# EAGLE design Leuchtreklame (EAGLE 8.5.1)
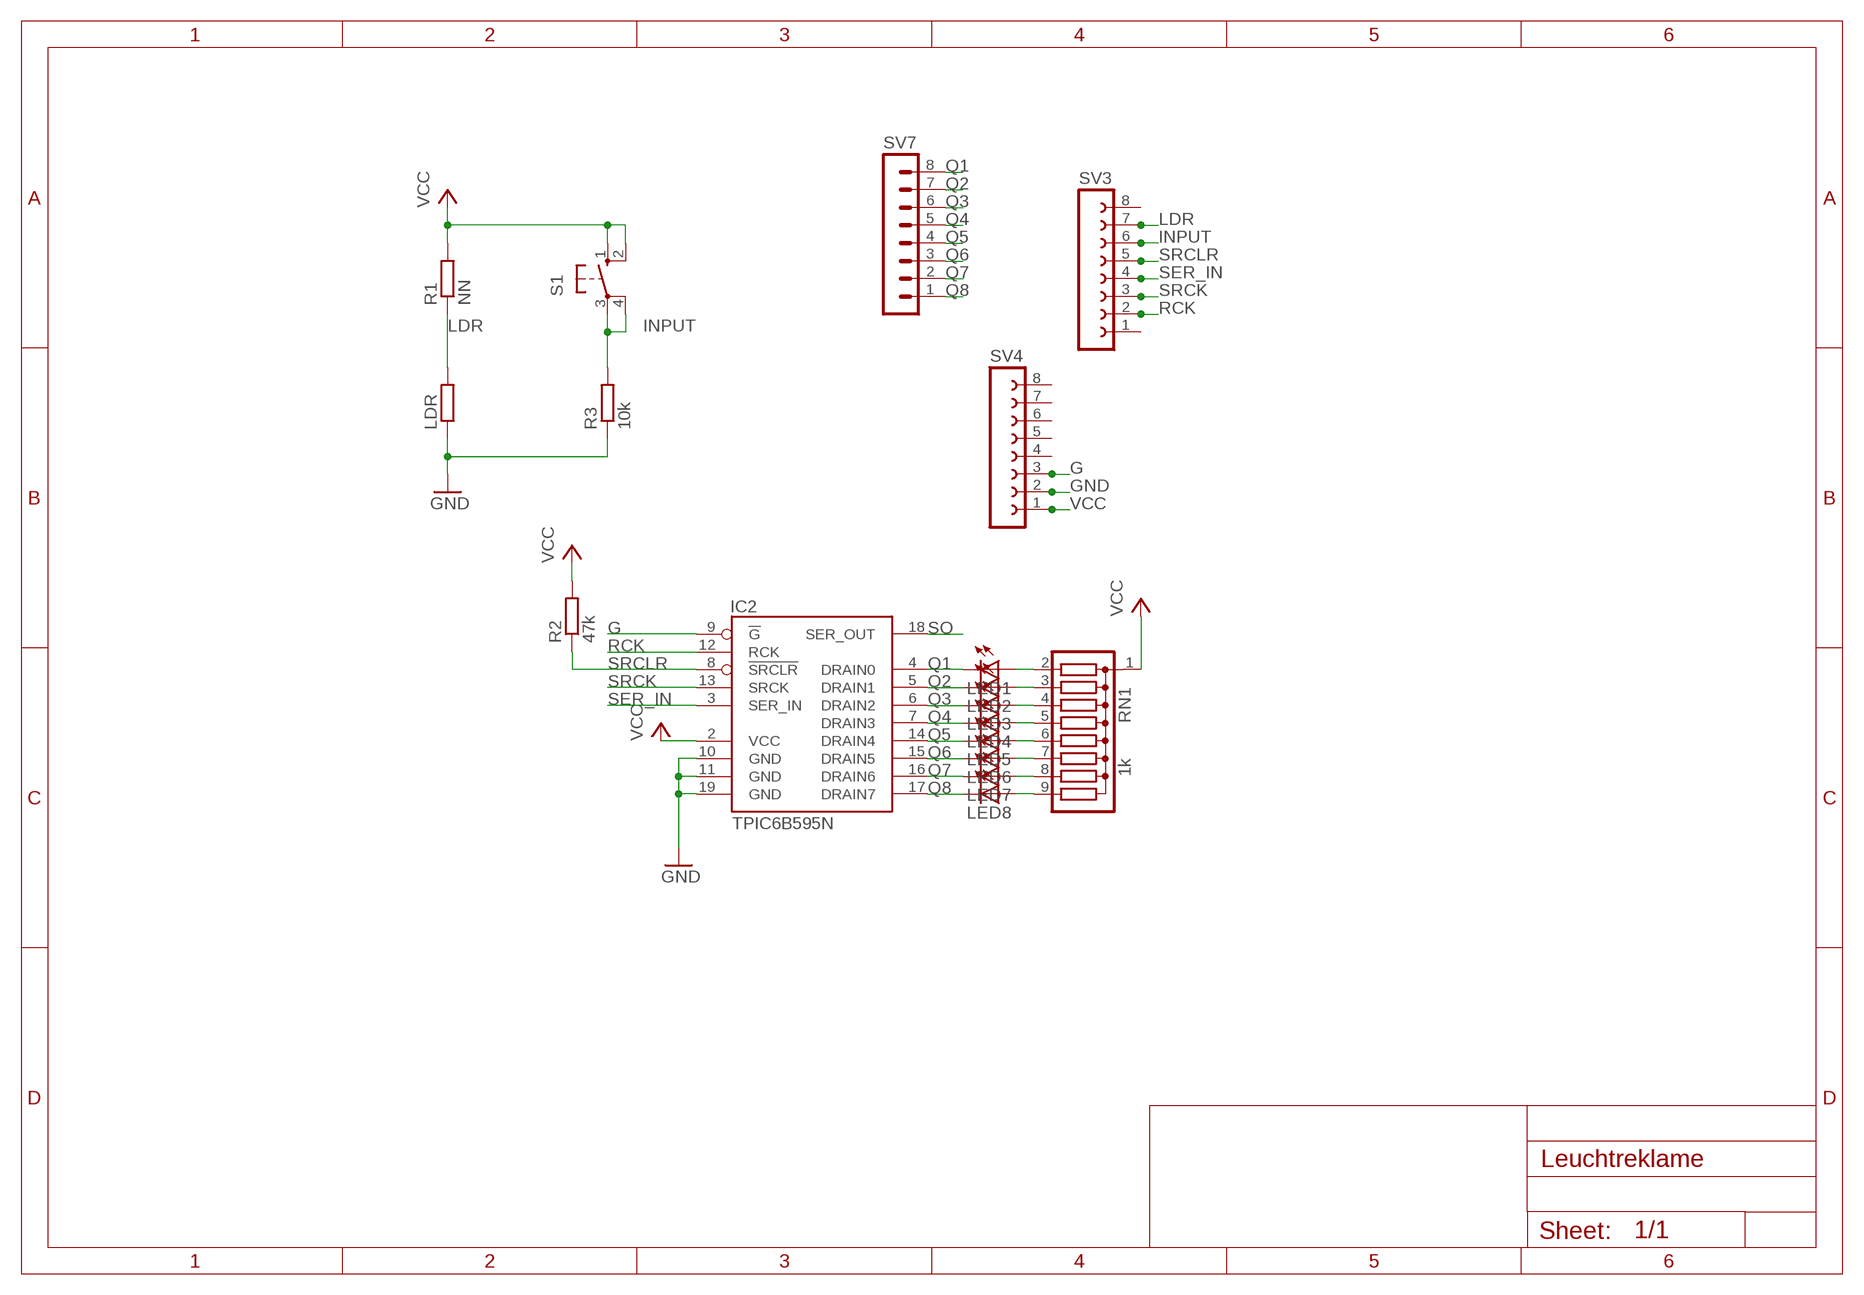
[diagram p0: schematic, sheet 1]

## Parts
IC2  TPIC6B595N  [DIL20]
LDR  R-EU_0204/5  [0204/5]
LED1  LEDSML0805  [SML0805]
LED2  LEDSML0805  [SML0805]
LED3  LEDSML0805  [SML0805]
LED4  LEDSML0805  [SML0805]
LED5  LEDSML0805  [SML0805]
LED6  LEDSML0805  [SML0805]
LED7  LEDSML0805  [SML0805]
LED8  LEDSML0805  [SML0805]
R1  NN  R-EU_0207/10  [0207/10]
R2  47k  R-EU_0207/10  [0207/10]
R3  10k  R-EU_0207/10  [0207/10]
RN1  1k  G08R  [SIL9]
S1  10-XX  [B3F-10XX]
SV3  FE08-1  [FE08]
SV4  FE08-1  [FE08]
SV7  MA08-1  [MA08-1]

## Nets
G: IC2.9(!G) SV4.3
GND: IC2.10(GND) IC2.11(GND) IC2.19(GND) LDR.1 R3.1 SV4.2
INPUT: R3.2 S1.3(P) S1.4(P1) SV3.6
LDR: LDR.2 R1.1 SV3.7
N$2: LED1.A RN1.2
N$3: LED2.A RN1.3
N$5: LED3.A RN1.4
N$6: LED4.A RN1.5
N$7: LED5.A RN1.6
N$8: LED6.A RN1.7
N$9: LED7.A RN1.8
N$10: LED8.A RN1.9
Q1: IC2.4(DRAIN0) LED1.C SV7.8
Q2: IC2.5(DRAIN1) LED2.C SV7.7
Q3: IC2.6(DRAIN2) LED3.C SV7.6
Q4: IC2.7(DRAIN3) LED4.C SV7.5
Q5: IC2.14(DRAIN4) LED5.C SV7.4
Q6: IC2.15(DRAIN5) LED6.C SV7.3
Q7: IC2.16(DRAIN6) LED7.C SV7.2
Q8: IC2.17(DRAIN7) LED8.C SV7.1
RCK: IC2.12(RCK) SV3.2
SER_IN: IC2.3(SER_IN) SV3.4
SO: IC2.18(SER_OUT)
SRCK: IC2.13(SRCK) SV3.3
SRCLR: IC2.8(!SRCLR) R2.1 SV3.5
VCC: IC2.2(VCC) R1.2 R2.2 RN1.1 S1.1(S) S1.2(S1) SV4.1
Unconnected: SV3.1 SV3.8 SV4.4 SV4.5 SV4.6 SV4.7 SV4.8

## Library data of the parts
IC2 = TPIC6B595:TPIC6B595
LDR R1-R3 = 1a BK_Hennef:R-EU_: RESISTOR, European symbol
LED1-LED8 = 1a BK_Hennef:LED: LED
RN1 = resistor-sil:G08R: SIL RESISTOR; OC_FARNELL: unknown; OC_NEWARK: unknown
S1 = switch-omron:10-XX: OMRON SWITCH; MPN: B3F-1000; OC_FARNELL: 176432; OC_NEWARK: 36M3542
SV3 SV4 = con-lsta:FE08-1: FEMALE HEADER; OC_FARNELL: unknown; OC_NEWARK: unknown
SV7 = con-lstb:MA08-1: PIN HEADER; OC_FARNELL: unknown; OC_NEWARK: unknown

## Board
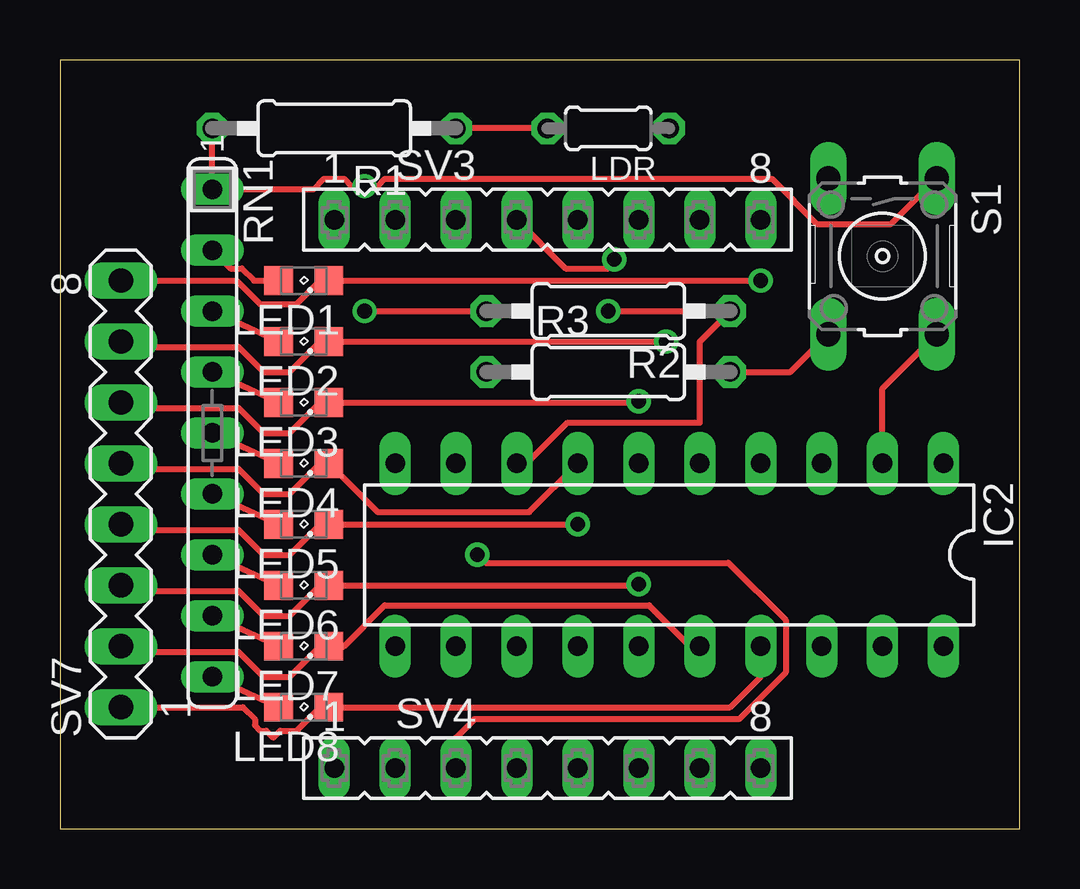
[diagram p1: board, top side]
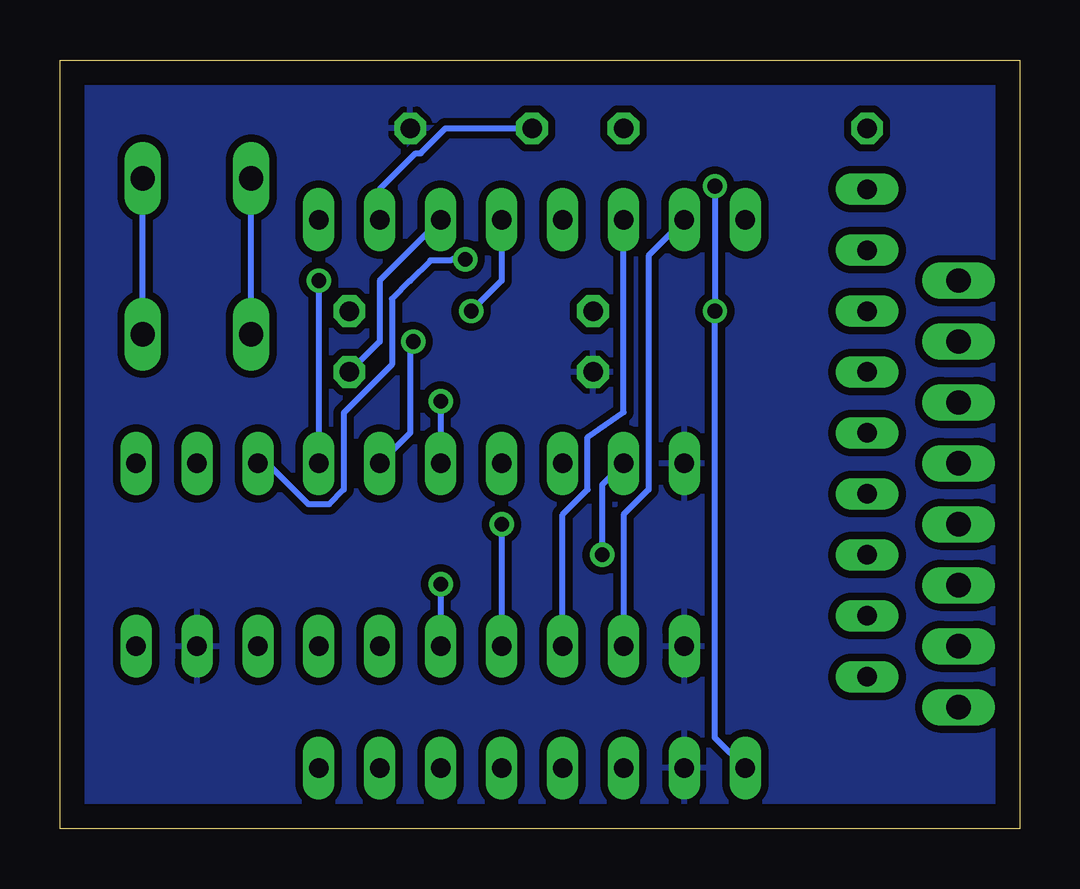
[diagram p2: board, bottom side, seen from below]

Size 40 x 32.06 mm. Coordinates in mm from the lower left corner, seen from the top.
Outline: 0,0 40,0 40,32.06 0,32.06 0,0
Copper layers (1*16): Top 0.035mm / dielectric 1.5mm / Bottom 0.035mm
Design rules "Bilex DRU": minimum track width 10mil, minimum drill 24mil, track to track 10mil, track to pad 10mil, pad to pad 10mil, via to via 10mil, smd to smd 10mil, copper to edge 40mil, drill to drill 8mil, minimum pad ring 10mil, minimum via ring 8mil, stop-mask expansion 4mil, vias tented up to drill 0mil, thermal gap 10mil

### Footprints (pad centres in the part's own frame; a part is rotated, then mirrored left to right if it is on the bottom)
DIL20 = drill 0.813 long: 1 -11.43,-3.81; 2 -8.89,-3.81; 3 -6.35,-3.81; 4 -3.81,-3.81; 5 -1.27,-3.81; 6 1.27,-3.81; 7 3.81,-3.81; 8 6.35,-3.81; 9 8.89,-3.81; 10 11.43,-3.81; 11 11.43,3.81; 12 8.89,3.81; 13 6.35,3.81; 14 3.81,3.81; 15 1.27,3.81; 16 -1.27,3.81; 17 -3.81,3.81; 18 -6.35,3.81; 19 -8.89,3.81; 20 -11.43,3.81
0204/5 = drill 0.813 octagon: 1 -2.54,0; 2 2.54,0
SML0805 = smd 1.2 x 1.2: A 1.05,0; C -1.05,0
0207/10 = drill 0.813 octagon: 1 -5.08,0; 2 5.08,0
SIL9 = drill 0.813 long: 1 -10.16,0; 2 -7.62,0; 3 -5.08,0; 4 -2.54,0; 5 0,0; 6 2.54,0; 7 5.08,0; 8 7.62,0; 9 10.16,0
B3F-10XX = drill 1.016 long: 1 -3.251,2.261; 2 3.251,2.261; 3 -3.251,-2.261; 4 3.251,-2.261
FE08 = drill 0.813 long: 1 -8.89,0; 2 -6.35,0; 3 -3.81,0; 4 -1.27,0; 5 1.27,0; 6 3.81,0; 7 6.35,0; 8 8.89,0
MA08-1 = drill 1.016 long: 1 -8.89,0; 2 -6.35,0; 3 -3.81,0; 4 -1.27,0; 5 1.27,0; 6 3.81,0; 7 6.35,0; 8 8.89,0

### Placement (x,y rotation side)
IC2  25.4,11.43 180 top
LDR  22.86,29.21 180 top
LED1  10.16,22.86 180 top
LED2  10.16,20.32 180 top
LED3  10.16,17.78 180 top
LED4  10.16,15.24 180 top
LED5  10.16,12.7 180 top
LED6  10.16,10.16 180 top
LED7  10.16,7.62 180 top
LED8  10.16,5.08 180 top
R1  11.43,29.21 180 top
R2  22.86,21.59 180 top
R3  22.86,19.05 0 top
RN1  6.35,16.51 270 top
S1  34.29,23.88 270 top
SV3  20.32,25.4 0 top
SV4  20.32,2.54 0 top
SV7  2.54,13.97 90 top

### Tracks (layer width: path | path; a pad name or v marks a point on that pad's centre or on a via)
G  (via drill 0.61)
  Top 0.254: v17.4,11.43 17.73,11.1 27.86,11.1 30.25,8.71 30.25,6.53 28.3,4.57 17.27,4.57 16.51,3.81 SV4.3
  Bottom 0.254: IC2.9 17.4,14.35 v17.4,11.43
GND
  pour Bottom (isolate 0.305): 0,32.06 0,0 40,0 40,32.06
INPUT
  Top 0.254: R3.2 30.45,19.05 S1.4
  Bottom 0.254: S1.4 S1.3 | SV3.6 26.67,22.86 26.67,20.32 R3.2
LDR
  Top 0.254: LDR.2 R1.1
  Bottom 0.254: SV3.7 26.67,26.67 25.17,28.17 24.97,28.17 23.93,29.21 LDR.2
N$2
  Top 0.254: RN1.2 7.11,23.37 7.58,23.37 8.09,22.86 LED1.A
N$3
  Top 0.254: RN1.3 LED2.A
N$5
  Top 0.254: RN1.4 LED3.A
N$6
  Top 0.254: RN1.5 LED4.A
N$7
  Top 0.254: RN1.6 LED5.A
N$8
  Top 0.254: LED6.A RN1.7
N$9
  Top 0.254: RN1.8 LED7.A
N$10
  Top 0.254: RN1.9 LED8.A
Q1  (via drill 0.61)
  Top 0.254: SV7.8 7.37,22.86 8.35,21.88 9.87,21.88 10.85,22.86 LED1.C 25.4,22.86 v29.21,22.86
  Bottom 0.254: v29.21,22.86 IC2.4
Q2  (via drill 0.61)
  Top 0.254: SV7.7 2.77,20.09 7.44,20.09 8.48,19.05 9.58,19.05 10.85,20.32 LED2.C v25.27,20.32
  Bottom 0.254: v25.27,20.32 25.4,20.19 25.4,16.51 IC2.5
Q3  (via drill 0.61)
  Top 0.254: SV7.6 2.77,17.55 7.44,17.55 8.48,16.51 9.58,16.51 10.85,17.78 LED3.C 24.08,17.78 v24.13,17.83
  Bottom 0.254: v24.13,17.83 IC2.6
Q4
  Top 0.254: SV7.5 2.77,15.01 7.44,15.01 8.48,13.97 9.58,13.97 10.85,15.24 LED4.C | 11.43,15.24 LED4.C | LED4.C 13.24,13.21 19.56,13.21 IC2.7
Q5  (via drill 0.61)
  Top 0.254: SV7.4 2.77,12.47 7.44,12.47 8.48,11.43 9.58,11.43 10.85,12.7 LED5.C v21.59,12.7
  Bottom 0.254: v21.59,12.7 IC2.14
Q6  (via drill 0.61)
  Top 0.254: SV7.3 2.77,9.93 7.44,9.93 8.48,8.89 9.58,8.89 10.85,10.16 LED6.C 24.08,10.16 v24.13,10.21
  Bottom 0.254: v24.13,10.21 IC2.15
Q7
  Top 0.254: SV7.2 2.77,7.39 7.44,7.39 8.48,6.35 9.58,6.35 10.85,7.62 LED7.C 11.84,7.62 13.54,9.32 24.56,9.32 26.26,7.62 IC2.16
Q8
  Top 0.254: SV7.1 7.62,5.08 8.13,4.57 8.13,4.32 8.35,4.1 8.6,4.1 8.89,3.81 9.18,4.1 9.87,4.1 10.85,5.08 LED8.C 27.94,5.08 29.21,6.35 IC2.17
RCK
  Bottom 0.254: IC2.12 16.51,13.11 15.47,14.15 15.47,23.9 SV3.2
SER_IN  (via drill 0.61)
  Top 0.254: SV3.4 21.08,23.37 22.86,23.37 23.11,23.62 v23.11,23.75
  Bottom 0.254: v23.11,23.75 23.65,23.75 23.7,23.7 24.56,23.7 25.4,22.86 26.16,22.1 26.16,19.36 28.17,17.35 28.17,14.15 28.78,13.54 29.64,13.54 31.34,15.24 IC2.3
SRCK
  Bottom 0.254: IC2.13 19.05,13.11 18.01,14.15 18.01,16.33 16.51,17.37 SV3.3
SRCLR  (via drill 0.61)
  Top 0.254: IC2.8 19.46,15.24 21.16,16.94 26.67,16.94 26.67,20.32 R2.1 v22.86,21.59
  Bottom 0.254: SV3.5 21.59,22.86 v22.86,21.59
VCC  (via drill 0.61)
  Top 0.254: IC2.2 34.29,18.36 S1.2 | S1.1 34.65,25.22 31.56,25.22 29.68,27.1 13.54,27.1 13.24,26.8 v12.7,26.8 12.16,26.8 11.86,27.1 11,27.1 10.57,26.67 RN1.1 R1.2 | v12.7,21.59 R2.2
  Bottom 0.254: S1.2 S1.1 | SV4.1 12.7,3.81 v12.7,21.59 v12.7,26.8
